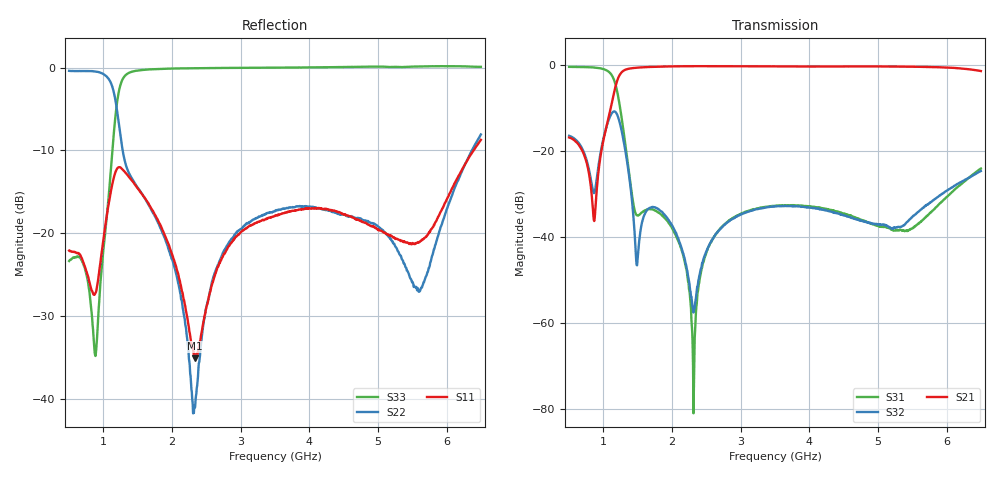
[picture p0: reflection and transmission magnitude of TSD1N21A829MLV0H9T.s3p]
# MHZ S RI R 50
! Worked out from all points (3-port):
!   1001 points, 500 MHz to 6.5 GHz, reference 50 ohm
!   strongest paths, dB at 500 MHz, 2 GHz, 3.5 GHz, 5 GHz, 6.5 GHz:
!     S21: -16.8, -0.2, -0.2, -0.2, -1.3
!     S32: -16.4, -37.2, -32.8, -36.9, -24.6
!     S31: -0.3, -37.9, -32.7, -37.3, -24.0
!   lowest |S11| = -35.1 dB at 2.33 GHz (marker M1), VSWR 1.04, Z = 48.4 - j0.558 ohm
!   |S11| at or under -10 dB: start of sweep to 6.393 GHz
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500  -0.0758 -0.0198  0.1299 0.066  0.5135 -0.8132
     0.1294 0.0658  -0.399 -0.8713  0.1419 -0.0528
     0.5153 -0.8123  0.1425 -0.0528  -0.027 -0.0622
866  -0.0423 0.00676  -0.000212 -0.0155  -0.4106 -0.8534
     -0.000268 -0.0155  -0.9518 -0.0404  0.0298 -0.0138
     -0.4099 -0.8524  0.03 -0.0137  -0.0196 0.00568
1124  -0.0301 0.1906  -0.3628 0.0862  -0.7324 0.2169
      -0.3623 0.0877  -0.4308 0.651  0.1533 -0.2329
      -0.7317 0.2182  0.1541 -0.2328  0.2048 0.2083
1484  -0.1313 -0.1376  0.1878 0.9202  -0.016 0.00853
      0.1883 0.9213  -0.0795 0.1757  0.00244 0.00426
      -0.0161 0.0086  0.00239 0.00415  0.4362 -0.8559
2072  -0.0531 0.0271  0.8048 0.552  -0.00871 -0.0045
      0.8043 0.5525  -0.0115 0.0527  -0.000338 -0.0106
      -0.00866 -0.00454  -0.000327 -0.0105  -0.3014 -0.9441
2330  -0.0165 -0.00576  0.9005 0.3865  0.000465 0.000123
      0.9004 0.3862  0.0088 0.000507  0.00165 -6.97e-06
      0.000613 0.000278  0.00153 2.84e-05  -0.4442 -0.8897
2582  -0.00285 -0.0488  0.9496 0.238  0.00898 0.0026
      0.95 0.2373  0.0191 -0.0471  0.00678 0.00661
      0.00889 0.0025  0.0067 0.00656  -0.5402 -0.8374
3500  -0.0383 -0.1211  0.9538 -0.1988  0.0232 0.000122
      0.9544 -0.1984  -0.0103 -0.1353  0.0212 0.00872
      0.0232 0.000111  0.0213 0.00862  -0.7527 -0.6614
5600  0.0285 -0.0834  0.3506 -0.8992  -0.00983 -0.0109
      0.3477 -0.8978  -0.0149 0.0417  0.00859 0.0185
      -0.00964 -0.0109  0.00837 0.0184  -0.9792 -0.2821
6500  0.2745 -0.2431  -0.2781 -0.8166  -0.0634 -0.00149
      -0.2799 -0.8136  0.3883 -0.0736  0.0421 0.0416
      -0.0632 -0.00171  0.0418 0.0419  -1.001 -0.1629
